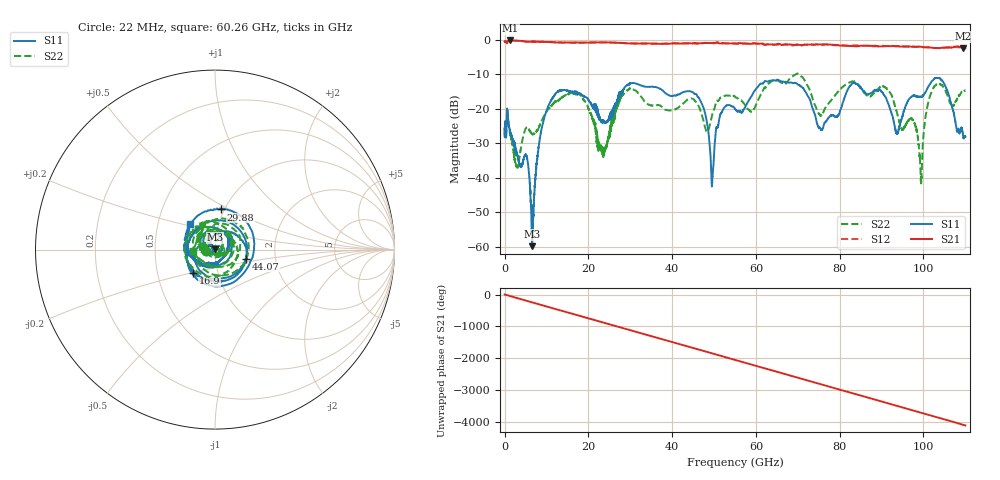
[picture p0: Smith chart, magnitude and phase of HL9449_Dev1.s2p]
! 5/9/2022 12:32:21 PM
! C:\USERS\VECTORSTARUSER\DESKTOP\JASON\HL9449-11\HL9449-11-NE01.S2P
! CHANNEL.1
! TR.MEASUREMENT
! CORRECTED.DATA
# GHZ S RI R 50.0
! FREQ.GHZ  S11RE  S11IM  S21RE  S21IM  S12RE  S12IM  S22RE  S22IM
!; PortSelection: Port_12
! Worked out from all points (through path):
!   5000 points, 22 MHz to 110 GHz, reference 50 ohm
!   highest |S21| = -0.26 dB at 1.386 GHz (marker M1); lowest = -2.5 dB at 109.5 GHz (marker M2)
!   group delay of S21, straight-line fit = 103 ps
!   lowest |S11| = -59.8 dB at 6.6 GHz (marker M3), VSWR 1.00, Z = 50 + j0.102 ohm
!   |S11| at or under -10 dB: start of sweep to end of sweep
!   |S22| runs from -41.6 to -9.8 dB; largest |S21 - S12| = 0.046
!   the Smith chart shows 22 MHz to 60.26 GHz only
!   S11 on the Smith chart (normalised r, x): 22 MHz: 0.90, -0.01; 16.9 GHz: 0.76, -0.21; 29.88 GHz: 0.96, +0.45; 44.07 GHz: 1.41, -0.14; 60.26 GHz: 0.73, +0.22
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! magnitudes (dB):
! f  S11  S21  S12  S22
! 22 MHz  -25.6  -0.5  -0.5  -25.5
! 1.386 GHz  -27.0  -0.3  -0.3  -27.8
! 3.014 GHz  -33.1  -0.3  -0.4  -37.0
! 5.302 GHz  -33.9  -0.6  -0.6  -25.4
! 6.6 GHz  -59.8  -0.6  -0.6  -27.4
! 10.1 GHz  -20.3  -0.7  -0.7  -20.7
! 16.9 GHz  -15.0  -0.8  -0.9  -15.4
! 18.37 GHz  -16.0  -0.9  -0.9  -16.5
! 23.65 GHz  -23.6  -0.8  -0.8  -33.3
! 29.88 GHz  -12.9  -1.1  -1.1  -14.3
! 36.7 GHz  -14.0  -1.2  -1.2  -19.0
! 44.07 GHz  -14.9  -1.1  -1.1  -17.2
! 49.54 GHz  -41.6  -1.0  -1.0  -21.8
! 51.79 GHz  -21.1  -1.1  -1.2  -16.7
! 55.02 GHz  -20.1  -1.1  -1.2  -16.5
! 60.26 GHz  -13.9  -1.2  -1.2  -18.3
! 73.35 GHz  -19.3  -1.5  -1.4  -16.3
! 91.67 GHz  -18.8  -1.9  -1.8  -14.7
! 99.33 GHz  -16.6  -2.1  -2.1  -38.5
! 102.4 GHz  -11.5  -2.4  -2.4  -13.8
! 109.5 GHz  -28.4  -2.5  -2.5  -14.9
! 110 GHz  -28.1  -2.5  -2.5  -14.7
